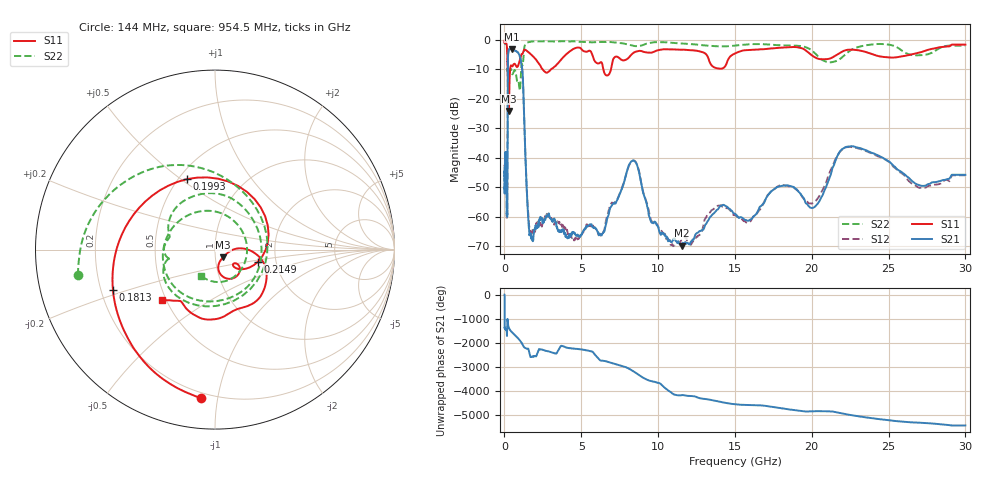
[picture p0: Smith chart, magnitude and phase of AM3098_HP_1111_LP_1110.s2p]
! Date/Time: Thu, Feb 28, 2019 8:48 AM
! Network Analyzer: Agilent Technologies E8364B Rev: A.07.50.67
! Sweep from 0.010 to 30.000 GHz, 1601 Points, Sweep Type: LOG
! Power Supply: 5.023 V, 0.002 A
# Hz S DB R 50
!freq MagS11 AngS11 MagS21 AngS21 MagS12 AngS12 MagS22 AngS22
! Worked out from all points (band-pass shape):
!   1601 points, 10 MHz to 30 GHz, reference 50 ohm
!   highest |S21| = -3.13 dB at 495.6 MHz (marker M1); lowest = -69.9 dB at 11.54 GHz (marker M2)
!   |S21| within 3 dB of the highest: 228.4 MHz to 1.028 GHz (799.5 MHz wide, 127 % of centre)
!   lowest |S11| = -24.2 dB at 293 MHz (marker M3), VSWR 1.13, Z = 54.6 - j4.59 ohm
!   |S11| at or under -10 dB: 210.1 MHz to 370.8 MHz (160.7 MHz wide, 55.3 % of centre); 2.474 GHz to 3.04 GHz (565.4 MHz wide, 20.5 % of centre); 6.435 GHz to 6.933 GHz (497.8 MHz wide, 7.45 % of centre)
!   |S22| runs from -17.2 to -0.5 dB; largest |S21 - S12| = 0.012
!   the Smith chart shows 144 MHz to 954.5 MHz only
!   S11 on the Smith chart (normalised r, x): 144 MHz: 0.17, -0.90; 181.3 MHz: 0.25, -0.18; 199.3 MHz: 0.55, +0.53; 214.9 MHz: 1.61, -0.23; 954.5 MHz: 0.47, -0.32
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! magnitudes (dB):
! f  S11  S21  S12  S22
! 10 MHz  -0.3  -45.1  -42.8  -0.6
! 16.01 MHz  -1.1  -49.9  -51.2  -1.3
! 38.04 MHz  -0.2  -40.6  -40.8  -0.8
! 101.4 MHz  -0.9  -39.9  -39.6  -1.6
! 144 MHz  -1.6  -53.6  -54.3  -2.2
! 144.7 MHz  -1.6  -53.8  -55.8  -2.2
! 181.3 MHz  -4.3  -59.8  -57.0  -5.5
! 199.3 MHz  -7.5  -34.6  -34.7  -10.7
! 214.9 MHz  -12.1  -11.9  -11.9  -9.5
! 293 MHz  -24.2  -3.3  -3.3  -11.5
! 495.6 MHz  -9.0  -3.1  -3.1  -11.6
! 550.5 MHz  -8.7  -3.3  -3.3  -11.4
! 954.5 MHz  -7.8  -5.0  -5.0  -15.6
! 1.19 GHz  -4.6  -12.3  -12.3  -8.5
! 1.606 GHz  -4.4  -64.4  -63.1  -0.8
! 2.084 GHz  -6.9  -63.9  -62.2  -0.5
! 6.265 GHz  -7.6  -66.0  -66.5  -0.7
! 7.926 GHz  -6.7  -45.5  -45.5  -1.5
! 11.54 GHz  -3.4  -69.9  -67.9  -1.3
! 20.2 GHz  -6.0  -56.7  -55.0  -4.6
! 22.56 GHz  -3.4  -36.1  -36.4  -3.5
! 30 GHz  -1.7  -45.8  -46.0  -2.0
